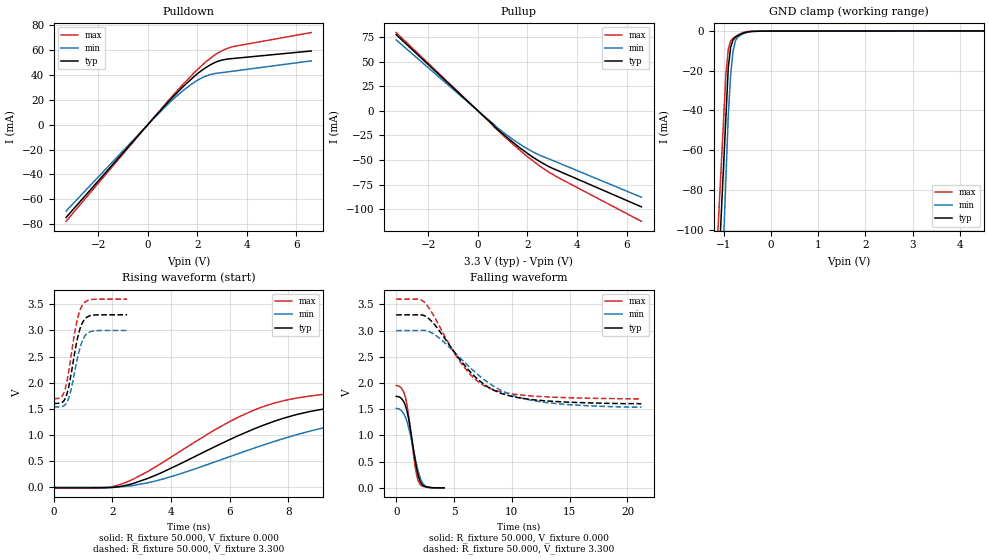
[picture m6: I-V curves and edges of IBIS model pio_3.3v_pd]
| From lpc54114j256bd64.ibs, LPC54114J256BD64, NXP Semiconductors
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[Model]   pio_3.3v_pd
Model_type I/O
Vinl=8.000E-01
Vinh=2.000E+00
Vref=0.000E+00
Rref=1.000E+06
Cref=2.000E-11
Vmeas=1.650E+00
C_comp   9.060E-13   8.700E-13   9.240E-13
[Voltage Range]   3.300E+00   3.000E+00   3.600E+00
[POWER Clamp Reference]   3.300E+00   3.000E+00   3.600E+00
[GND Clamp Reference]   0.000E+00   0.000E+00   0.000E+00
[Pullup Reference]   3.300E+00   3.000E+00   3.600E+00
[Pulldown Reference]   0.000E+00   0.000E+00   0.000E+00
[Temperature Range]   25   105   -40
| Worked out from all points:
|   slope of the pulldown table from 0 to 0.495 V, typ, clamps not added: 44.8 ohm
|   slope of the pullup table from 0 to 0.495 V, typ, clamps not added: 43.6 ohm
|   GND clamp passes 1 mA (typ) near -0.58 V on its own axis
|   rising waveform, R_fixture 50.000, V_fixture 0.000: 20-80 % time 4.35ns typ, 5.29ns min, 3.74ns max; typ from -0.012 V to 1.73 V
|   falling waveform, R_fixture 50.000, V_fixture 0.000: 20-80 % time 788ps typ, 920ps min, 704ps max; typ from 1.74 V to 0.001 V
|   rising waveform, R_fixture 50.000, V_fixture 3.300: 20-80 % time 341ps typ, 343ps min, 341ps max; typ from 1.6 V to 3.3 V
|   falling waveform, R_fixture 50.000, V_fixture 3.300: 20-80 % time 3.95ns typ, 4.88ns min, 3.41ns max; typ from 3.3 V to 1.6 V
[GND Clamp]
-3.3V     -1.216A    -1.571A    -1.123A
-950mV    -43.37mA   -74.42mA   -21.6mA
-900mV    -18.43mA   -42.58mA   -9.201mA
-850mV    -8.133mA   -22.12mA   -4.954mA
-800mV    -4.528mA   -10.24mA   -3.565mA
-750mV    -3.154mA   -4.987mA   -2.774mA
-700mV    -2.303mA   -3.029mA   -1.982mA
-600mV    -1.145mA   -1.463mA   -880.3uA
-400mV    -198.5uA   -152.7uA   -64.24uA
-200mV    -33.8uA    -31.76uA   -14.46uA
6.6V      135.5uA    140.2uA    126.4uA
[Power Clamp]
-3.3V     0A         0A         0A
0V        0A         0A         0A
3.3V      0A         0A         0A
6.6V      0A         0A         0A
[Pullup]
-3.3V     77.49mA    72.2mA     79.65mA
760mV     -18.12mA   -16.61mA   -18.86mA
1.46V     -32.91mA   -29.95mA   -34.98mA
2.12V     -45.48mA   -40.34mA   -48.91mA
2.58V     -52.8mA    -46.08mA   -57.61mA
3.14V     -59.87mA   -51.73mA   -66.48mA
6.6V      -97.67mA   -87.89mA   -112.4mA
[Pulldown]
-3.3V     -74.59mA   -69.4mA    -77.67mA
140mV     3.186mA    2.948mA    3.327mA
940mV     20.73mA    18.9mA     21.9mA
1.44V     30.86mA    27.69mA    32.8mA
1.78V     37.07mA    32.83mA    39.81mA
2.24V     44.5mA     38.17mA    48.65mA
2.78V     50.6mA     41.38mA    57.01mA
3.34V     53.01mA    42.75mA    62.23mA
6.6V      59.25mA    51.3mA     74.05mA
[Rising Waveform]
R_fixture = 50.000
V_fixture = 0.000
V_fixture_min = 0.000
V_fixture_max = 0.000
|  time   V(typ)   V(min)   V(max)
0s        -11.6mV    650.1uV    -11.05mV
1.75ns    -10.32mV   317.2uV    -6.202mV
2.35ns    23.6mV     12.5mV     69.84mV
3.7ns     286.1mV    154.2mV    469.2mV
6.3ns     989.1mV    644.9mV    1.343V
7.3ns     1.218V     836.1mV    1.572V
8.35ns    1.4V       1.016V     1.713V
10.15ns   1.565V     1.242V     1.825V
12.4ns    1.651V     1.384V     1.884V
20.7ns    1.733V     1.516V     1.939V
[Falling Waveform]
R_fixture = 50.000
V_fixture = 0.000
V_fixture_min = 0.000
V_fixture_max = 0.000
|  time   V(typ)   V(min)   V(max)
0s        1.744V     1.516V     1.952V
450ps     1.704V     1.472V     1.901V
800ps     1.565V     1.346V     1.721V
1.1ns     1.286V     1.129V     1.337V
1.65ns    518.7mV    555.1mV    392.1mV
1.8ns     339.4mV    407.6mV    218.5mV
1.95ns    201.7mV    280.3mV    112.8mV
2.2ns     75.16mV    127mV      42.9mV
2.55ns    23.87mV    32.14mV    15.45mV
4.15ns    673.6uV    650.1uV    235.6uV
[Rising Waveform]
R_fixture = 50.000
V_fixture = 3.300
V_fixture_min = 3.000
V_fixture_max = 3.600
|  time   V(typ)   V(min)   V(max)
0s        1.605V     1.538V     1.697V
250ps     1.615V     1.542V     1.724V
400ps     1.711V     1.584V     1.907V
550ps     2.039V     1.781V     2.367V
750ps     2.691V     2.319V     3.076V
850ps     2.949V     2.579V     3.315V
1ns       3.174V     2.835V     3.506V
1.15ns    3.262V     2.948V     3.573V
1.3ns     3.29V      2.985V     3.593V
2.5ns     3.3V       3V         3.6V
[Falling Waveform]
R_fixture = 50.000
V_fixture = 3.300
V_fixture_min = 3.000
V_fixture_max = 3.600
|  time   V(typ)   V(min)   V(max)
0s        3.3V       3V         3.6V
2.4ns     3.287V     3.004V     3.548V
3.45ns    3.078V     2.905V     3.202V
4.85ns    2.646V     2.628V     2.635V
5.8ns     2.365V     2.418V     2.323V
6.9ns     2.102V     2.191V     2.059V
8.15ns    1.896V     1.979V     1.894V
9.75ns    1.758V     1.791V     1.802V
12.1ns    1.675V     1.655V     1.747V
21.2ns    1.605V     1.538V     1.697V
[Ramp]
dV/dt_r   1.0470E+00/4.3389E-09   9.0819E-01/5.2888E-09   1.1703E+00/3.7398E-09
dV/dt_f   1.0173E+00/3.9512E-09   8.7689E-01/4.8527E-09   1.1419E+00/3.3989E-09
R_load = 50
